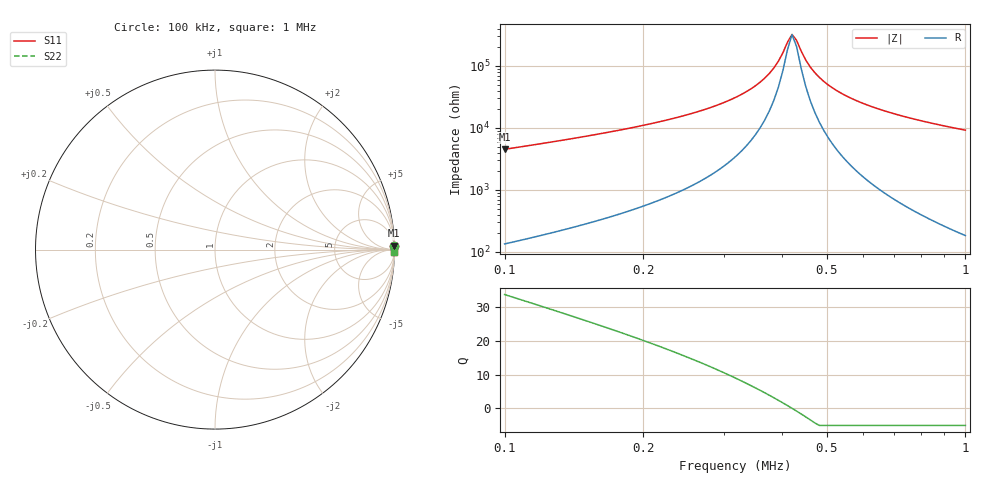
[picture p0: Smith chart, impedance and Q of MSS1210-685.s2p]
# MHz S MA R 50
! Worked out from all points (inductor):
!   102 points, 100 kHz to 1 MHz, reference 50 ohm
!   read as one part in series: L = 6.79 mH near 100 kHz
!   highest Q = 33.6 at 100 kHz (marker M1), where L = 7.2 mH
!   self-resonance near 420.5 kHz
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0.1  0.9991 1.3  0.02207 -87.0  0.02207 -87.0  0.9991 1.3
0.1507363  0.9994 0.8  0.01354 -87.0  0.01354 -87.0  0.9994 0.8
0.2546482  0.9996 0.3  0.005842 -85.8  0.005842 -85.8  0.9996 0.3
0.3126436  0.9996 0.2  0.003379 -83.7  0.003379 -83.7  0.9996 0.2
0.3503922  0.9997 0.1  0.002084 -80.5  0.002084 -80.5  0.9997 0.1
0.3667384  0.9997 0.1  0.001578 -77.8  0.001578 -77.8  0.9997 0.1
0.3838472  0.9997 0.1  0.001082 -72.5  0.001082 -72.5  0.9997 0.1
0.3926986  0.9997 0.0  0.000842 -67.6  0.000842 -67.6  0.9997 0.0
0.4017542  0.9997 0.0  0.0006131 -58.8  0.0006131 -58.8  0.9997 0.0
0.4110185  0.9997 0.0  0.0004147 -40.8  0.0004147 -40.8  0.9997 0.0
0.4204965  0.9997 0.0  0.0003107 -3.3  0.0003107 -3.3  0.9997 0.0
0.430193  0.9997 -0.0  0.0003867 37.5  0.0003867 37.5  0.9997 -0.0
0.4401132  0.9997 -0.0  0.0005754 58.1  0.0005754 58.1  0.9997 -0.0
0.4502621  0.9997 -0.0  0.0008009 67.9  0.0008009 67.9  0.9997 -0.0
0.460645  0.9997 -0.1  0.00104 73.4  0.00104 73.4  0.9997 -0.1
0.4712673  0.9997 -0.1  0.001285 76.7  0.001285 76.7  0.9997 -0.1
0.5046268  0.9997 -0.1  0.002039 81.9  0.002039 81.9  0.9997 -0.1
0.5528079  0.9997 -0.2  0.003071 84.7  0.003071 84.7  0.9997 -0.2
0.6195541  0.9997 -0.3  0.004403 86.4  0.004403 86.4  0.9997 -0.3
0.7103709  0.9997 -0.3  0.006081 87.3  0.006081 87.3  0.9997 -0.3
0.8524974  0.9997 -0.5  0.008503 88.0  0.008503 88.0  0.9997 -0.5
1  0.9997 -0.6  0.01085 88.2  0.01085 88.2  0.9997 -0.6
